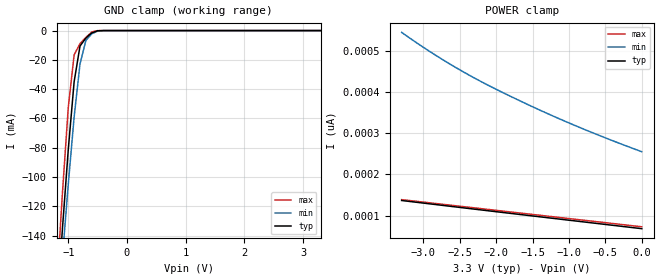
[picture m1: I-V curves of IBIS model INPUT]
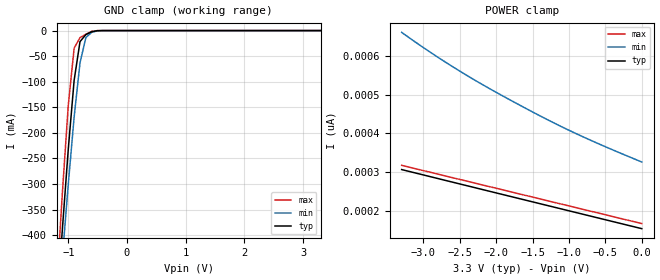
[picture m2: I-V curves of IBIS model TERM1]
|   PERICOM SEMICONDUCTOR CORP
|   IBIS Model of PI3C3306
|   Product Family: 3C
|   MSOP (U) Package
[IBIS Ver] 3.2
[Comment char] |_char
[File Name] pi3c3306_u_33v.ibs
[File Rev] 1.0
[Source] File originated at Pericom Semiconductor Corp.
[Date] 12/25/17
[Disclaimer] (C) Copyright PERICOM Semiconductor Corporation
   All rights reserved
  Pericom Semiconductor Corporation hereby grants the user of
  this IBIS model a non-exclusive, nontransferable license to
  use this IBIS model under the following terms.
  This IBIS model is provided on an "AS IS" basis and Pericom
  makes absolutely no warranty with respect to the information
  contained herein. PERICOM DISCLAIMS AND CUSTOMER WAIVES ALL
  WARRANTIES, EXPRESSED OR IMPLIED, INCLUDING WARRANTIES OF
  MERCHANTABILITY OR FITNESS FOR A PARTICULAR PURPOSE. The
  entire risk as to quality and performance is with the customer.
  Accordingly, in no event shall the company be liable for any
  damages, whether in contract or tort, including any lost
  profits or other incidental, consequential, exemplary, or
  punitive damages arising out of the use or application of the
  IBIS model provided in this package. Further, Pericom reserves
  the right to make changes without notice to any product herein
  to improve reliability, function, or design. Pericom does not
  convey any license under patent rights or any other intellectual
  property rights, including those of third parties.
  The user is granted this license only to use the IBIS model
  and is not granted rights to sell, load, rent, lease or license
  the IBIS model in whole or in part, or in modified form to anyone
  other than user. User may modify the IBIS model to suit its specific
  application but rights to derivative works and such modifications
  shall belong to Pericom.
  Pericom is not obligated to provide maintenance or support
  for the licensed IBIS model.
  Contact Pericom at ATTN: APPLICATION ENGINEERING / IBIS MODELS
  2380 Bering Drive, San Jose, CA 95131
[Component] PI3C3306
[Manufacturer] Pericom Semiconductor Corp.
[Package]
| variable   typ   min   max
R_pkg   0.04200   0.03995   0.04405
L_pkg   2.30669n   2.21200n   2.40138n
C_pkg   0.21108p   0.20715p   0.21500p
[Pin] signal_name  model_name   R_pin   L_pin   C_pin
1   _BE1   INPUT   0.04405   2.40138n   0.21500p
2   A1   TERM1   0.03995   2.21200n   0.20715p
3   B1   TERM2   0.03995   2.21200n   0.20715p
4   GND   GND   0.04405   2.40138n   0.21500p
5   A2   TERM1   0.04405   2.40138n   0.21500p
6   B2   TERM2   0.03995   2.21200n   0.20715p
7   _BE2   INPUT   0.03995   2.21200n   0.20715p
8   VCC   POWER   0.04405   2.40138n   0.21500p
[Series Switch Groups]
On 1 /
Off 2 /
[Series Pin Mapping]   pin_2   model_name  function_table_group
2   3   SWITCH1   1
5   6   SWITCH1   2
|   Model SWITCH1
[Model] SWITCH1
Model_type Series_switch
| variable   typ   min   max
C_comp   10.000pF   9.800pF   10.200pF
[Voltage Range]   3.3000V   2.9700V   3.6300V
[GND Clamp Reference]   0.0000V   0.0000V   0.0000V
[POWER Clamp Reference]   3.3000V   2.9700V   3.6300V
[Temperature Range]   25   85   -40
[On]
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[OFF]
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| Models and submodels in the file (4): INPUT (Input), SWITCH1 (Series_switch), TERM1 (Terminator), TERM2 (Terminator)
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|   Model INPUT
[Model] INPUT
Model_type Input
Vinl = 800mV
Vinh = 2.0V
| variable   typ   min   max
C_comp   3.500pF   3.400pF   3.600pF
[Voltage Range]   3.3000V   2.9700V   3.6300V
[GND Clamp Reference]   0.0000V   0.0000V   0.0000V
[POWER Clamp Reference]   3.3000V   2.9700V   3.6300V
[Temperature Range]   25   85   -40
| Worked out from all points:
|   GND clamp passes 1 mA (typ) near -0.56 V on its own axis
[GND Clamp]
| Voltage   I(typ)   I(min)   I(max)
-3.3V     -1.504A    -1.38A     -1.677A
-1.2V     -193.5mA   -207.1mA   -176.6mA
-1.1V     -135.8mA   -155mA     -111.4mA
-1V       -81.33mA   -105mA     -52.61mA
-900mV    -34.92mA   -59.01mA   -16.58mA
-800mV    -10.56mA   -22.8mA    -8.882mA
-700mV    -5.104mA   -6.74mA    -4.717mA
-600mV    -1.611mA   -2.212mA   -981.9uA
-500mV    -145.9uA   -381.4uA   -24.42uA
-400mV    -4.329uA   -29.72uA   -133.6nA
3.3V      68.04pA    277.2pA    66pA
[POWER Clamp]   |Note: Vtable = Vcc - Voutput
| Voltage   I(typ)   I(min)   I(max)
-3.3V     136.5pA    545.5pA    138.6pA
-3V       130.2pA    509pA      132.6pA
-2.7V     123.9pA    475.3pA    126.6pA
-2.4V     117.6pA    444.3pA    120.6pA
-2V       109.3pA    407.1pA    112.6pA
-1.5V     98.92pA    364.5pA    102.6pA
-1V       88.6pA     325.2pA    92.6pA
-500mV    78.3pA     288.9pA    82.6pA
0V        68.04pA    255.2pA    72.6pA
|   Model TERM1
[Model] TERM1
Model_type Terminator
| variable   typ   min   max
C_comp   5.000pF   4.900pF   5.100pF
[Voltage Range]   3.3000V   2.9700V   3.6300V
[GND Clamp Reference]   0.0000V   0.0000V   0.0000V
[POWER Clamp Reference]   3.3000V   2.9700V   3.6300V
[Temperature Range]   25   85   -40
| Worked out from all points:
|   GND clamp passes 1 mA (typ) near -0.54 V on its own axis
[GND Clamp]
| Voltage   I(typ)   I(min)   I(max)
-3.3V     -4.264A    -3.909A    -4.763A
-1.2V     -551.9mA   -590.4mA   -503.2mA
-1.1V     -387.8mA   -442.8mA   -316.8mA
-1V       -232.2mA   -300.6mA   -146.4mA
-900mV    -97.23mA   -169.1mA   -34.28mA
-800mV    -21.65mA   -63.17mA   -13.78mA
-700mV    -7.82mA    -13.64mA   -7.205mA
-600mV    -2.298mA   -3.355mA   -1.407mA
-400mV    -5.736uA   -40.64uA   -175.6nA
3.3V      153pA      351.8pA    151pA
[POWER Clamp]   |Note: Vtable = Vcc - Voutput
| Voltage   I(typ)   I(min)   I(max)
-3.3V     306.2pA    661.9pA    317.2pA
-2.9V     287.5pA    609.6pA    298.9pA
-2.5V     268.9pA    561.3pA    280.6pA
-2.1V     250.3pA    516.9pA    262.3pA
-1.7V     231.7pA    475.6pA    244pA
-1.3V     213.2pA    436pA      225.6pA
-900mV    194.6pA    399.2pA    207.3pA
-500mV    176.1pA    365.5pA    189pA
0V        153pA      325.8pA    166.1pA
